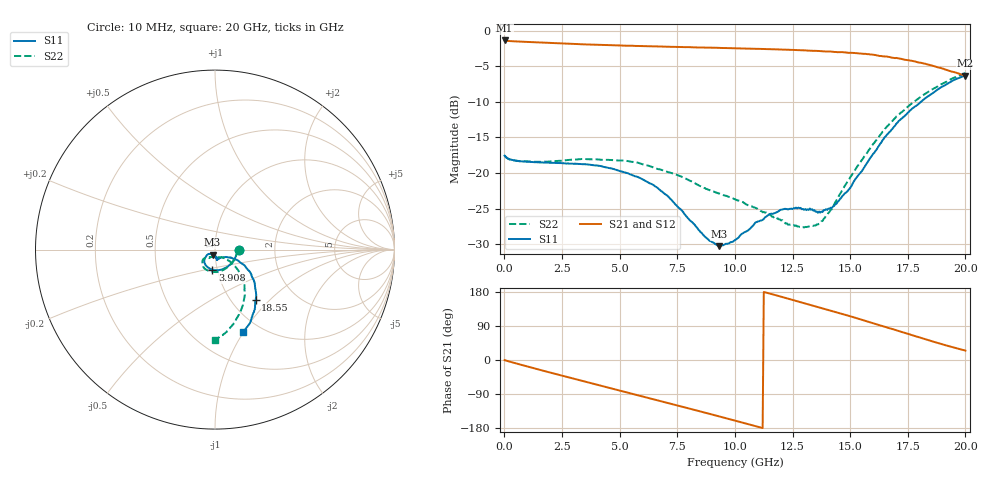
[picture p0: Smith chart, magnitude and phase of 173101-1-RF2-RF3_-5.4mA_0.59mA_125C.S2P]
!  2-Port S-parameters saved by WinCal
! VAR MeasName=S-Parameters (CALIBRATED_DATA) read from VNA (N5242A)
! VAR MeasDate=2017-7-20 10:54:35
! VAR NAME=173101-1-RF2-RF3_-5.4mA_0.59mA_125C
! VAR FILENAME=173101-1-RF2-RF3_-5.4mA_0.59mA_125C.S2P
! VAR DATE=2017-7-20 10:54:35
! VAR PHYS_PORTS=1,2
# Hz S DB R 50
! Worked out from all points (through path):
!   401 points, 10 MHz to 20 GHz, reference 50 ohm
!   highest |S21| = -1.39 dB at 10 MHz (marker M1); lowest = -6.3 dB at 20 GHz (marker M2)
!   group delay of S21, straight-line fit = 46.2 ps
!   lowest |S11| = -30.3 dB at 9.305 GHz (marker M3), VSWR 1.06, Z = 48.6 - j2.68 ohm
!   |S11| at or under -10 dB: start of sweep to 18.07 GHz
!   |S22| runs from -27.6 to -6.0 dB; largest |S21 - S12| = 0.0064
!   S11 on the Smith chart (normalised r, x): 10 MHz: 1.31, -0.01; 3.908 GHz: 0.95, -0.22; 18.55 GHz: 1.28, -0.83; 20 GHz: 0.83, -1.00
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1e7  -17.55 -1.1  -1.39 -0.2  -1.39 -0.2  -17.55 -1.1
1.559225e9  -18.51 -45.1  -1.69 -26.3  -1.70 -26.3  -18.43 -45.6
2.50875e9  -18.61 -68.3  -1.82 -41.5  -1.82 -41.5  -18.26 -68.2
3.358325e9  -18.74 -87.0  -1.93 -54.9  -1.93 -54.9  -18.02 -85.4
3.90805e9  -18.91 -97.1  -1.99 -63.5  -1.99 -63.5  -18.06 -94.6
5.357325e9  -20.03 -122.7  -2.13 -86.2  -2.14 -86.2  -18.33 -116.8
6.70665e9  -22.26 -137.5  -2.24 -107.4  -2.23 -107.4  -19.46 -130.5
7.956025e9  -26.30 -146.1  -2.32 -127.1  -2.35 -127.1  -20.92 -139.5
8.8056e9  -29.21 -136.5  -2.39 -140.6  -2.41 -140.6  -22.25 -140.8
9.30535e9  -30.26 -116.4  -2.43 -148.7  -2.43 -148.7  -22.87 -138.8
1.0005e10  -29.39 -90.9  -2.49 -160.0  -2.50 -160.0  -23.68 -135.3
1.090455e10  -26.90 -79.0  -2.56 -174.6  -2.57 -174.6  -24.91 -126.6
1.165418e10  -25.71 -79.3  -2.62 173.0  -2.63 173.0  -26.11 -121.5
1.24038e10  -25.02 -77.7  -2.71 160.4  -2.71 160.4  -27.25 -112.2
1.335332e10  -25.07 -71.2  -2.84 144.3  -2.81 144.3  -27.39 -84.8
1.38031e10  -25.46 -61.1  -2.92 136.4  -2.91 136.4  -26.71 -66.1
1.44028e10  -24.32 -45.1  -3.01 126.0  -3.04 126.1  -23.86 -45.3
1.555222e10  -19.51 -26.2  -3.26 105.3  -3.28 105.1  -17.99 -39.1
1.670165e10  -14.25 -29.0  -3.71 83.9  -3.77 83.7  -13.13 -46.3
1.76012e10  -11.20 -38.2  -4.21 67.4  -4.21 67.4  -10.40 -56.6
1.855072e10  -8.85 -51.2  -4.90 49.4  -4.97 49.6  -8.28 -69.7
2e10  -6.26 -71.1  -6.34 24.7  -6.39 25.3  -5.98 -89.9
